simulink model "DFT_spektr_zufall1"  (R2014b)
settings: Solver=ode45  StartTime=0.0  StopTime=10  RelTol=1e-3
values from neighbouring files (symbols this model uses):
  k = n    [fft_1.m]    (also in fft_2.m; fourier_reihe1.m; fourier_reihe_DFT_1.m = 0:nh; fourier_reihe_rechteck_1.m = 0:nh)
libraries: dspxfrm3 x1, dspstat3 x1

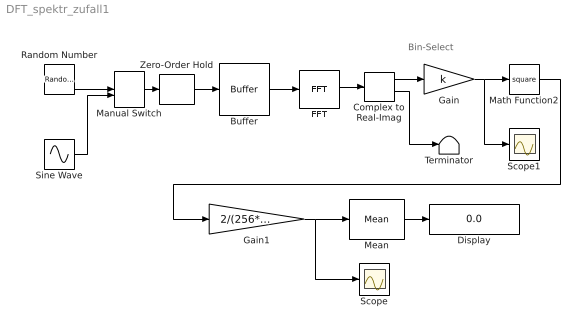
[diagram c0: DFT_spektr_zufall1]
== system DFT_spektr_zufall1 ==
  note: Bin-Select
  Buffer : Buffer  N=256  V=255  TreatMby1Signals=One channel
  Complex to Real-Imag : ComplexToRealImag
  Display : Display
  FFT : dspxfrm3/FFT  CompMethod=Table lookup  TableOpt=NEW  TableOptActive=Speed  BitRevOrder=off  InheritFFTLength=on  FFTLength=64  WrapInput=on  RowConvenienceOn=on  FFTImplementation=Auto  SkipNorm=off  firstCoeffDataTypeStr=Inherit: Same word length as input  firstCoeffLastDataTypeStr=Inherit: Same word length as input  outputMin=[]  outputMax=[]  roundingMode=Floor  overflowMode=off
  Gain : Gain  Gain=k  Multiplication=Matrix(K*u)
  Gain1 : Gain  Gain=2/(256*1000)
  Manual Switch : ManualSwitch
  Math Function2 : Math  Operator=square
  Mean : dspstat3/Mean  run=on  reset_popup=None  InputProcessing=Columns as channels (frame based)  directionMode=Each column  dimension=1  treatSBRowAsCol=on  roiEnable=off  roiType=Rectangles  roiPortion=Entire ROI  roiOutput=Individual statistics for each ROI  roiFlag=off  outputDataTypeStr=Inherit: Same as accumulator  outputLastDataTypeStr=Inherit: Same as accumulator  outputMin=[]  outputMax=[]  roundingMode=Floor  overflowMode=off
  Random Number : RandomNumber  SampleTime=1/1000
  Scope : Scope
  Scope1 : Scope
  Sine Wave : Sin  Frequency=2*pi*199.2188  SampleTime=1/1000
  Terminator : Terminator
  Zero-Order Hold : ZeroOrderHold  SampleTime=1/1000
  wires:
  Zero-Order Hold/1 -> Buffer/1
  Complex to Real-Imag/2 -> Terminator/1
  FFT/1 -> Complex to Real-Imag/1
  Complex to Real-Imag/1 -> Gain/1
  Gain/1 -> Scope1/1, Math Function2/1
  Math Function2/1 -> Gain1/1
  Mean/1 -> Display/1
  Gain1/1 -> Scope/1, Mean/1
  Manual Switch/1 -> Zero-Order Hold/1
  Random Number/1 -> Manual Switch/1
  Sine Wave/1 -> Manual Switch/2
  Buffer/1 -> FFT/1
